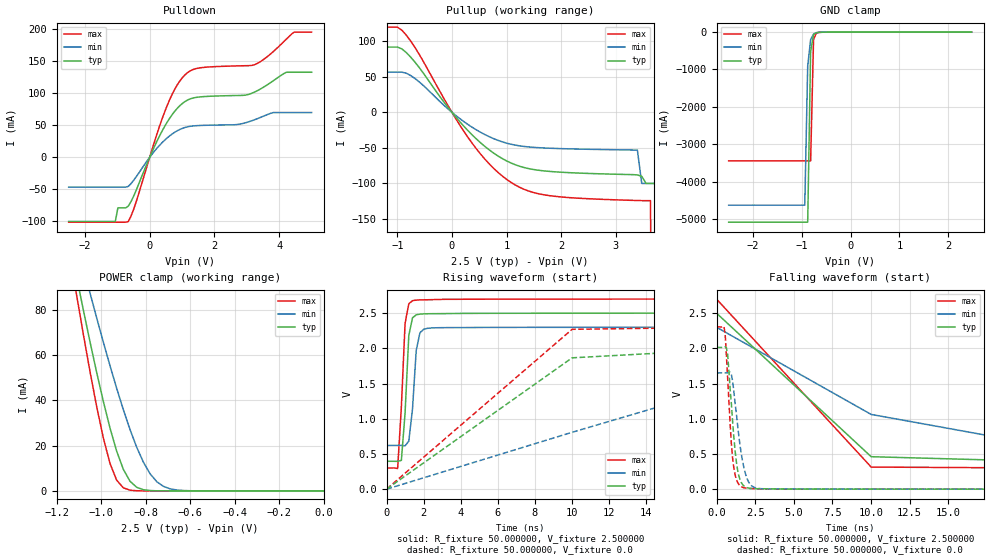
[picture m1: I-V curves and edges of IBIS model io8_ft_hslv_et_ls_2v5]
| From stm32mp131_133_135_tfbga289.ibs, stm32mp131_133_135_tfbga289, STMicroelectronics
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|   Model io8_ft_hslv_et_ls_2v5
[Model]  io8_ft_hslv_et_ls_2v5
Model_type I/O
Polarity   Non-Inverting
Enable   Active-Low
Vinl =   0.750000V
Vinh =   1.750000V
Vmeas =  1.250000V
Cref =   50.000000pF
Rref =   100.000000M
Vref =   0.0V
C_comp   3.268600pF   3.267200pF   3.310300pF
[Temperature Range]   25.000000   0.140000k   -40.000000
[Pullup Reference]   2.500000V   2.300000V   2.700000V
[Pulldown Reference]   0.0V   0.0V   0.0V
[POWER Clamp Reference]   2.500000V   2.300000V   2.700000V
[GND Clamp Reference]   0.0V   0.0V   0.0V
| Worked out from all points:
|   slope of the pulldown table from 0 to 0.375 V, typ, clamps not added: 9.35 ohm
|   slope of the pullup table from 0 to 0.375 V, typ, clamps not added: 11.7 ohm
|   GND clamp passes 1 mA (typ) near -0.47 V on its own axis
|   POWER clamp passes 1 mA (typ) near -0.82 V on its own axis
|   rising waveform, R_fixture 50.000000, V_fixture 2.500000: 20-80 % time 261ps typ, 279ps min, 266ps max; typ from 0.396 V to 2.5 V
|   rising waveform, R_fixture 50.000000, V_fixture 0.0: 20-80 % time 6.48ns typ, 12.5ns min, 6.1ns max; typ from 0 V to 2.01 V
|   falling waveform, R_fixture 50.000000, V_fixture 2.500000: 20-80 % time 6.2ns typ, 9.95ns min, 6.04ns max; typ from 2.5 V to 0.396 V
|   falling waveform, R_fixture 50.000000, V_fixture 0.0: 20-80 % time 452ps typ, 595ps min, 380ps max; typ from 2.01 V to 0 V
[Pulldown]
|Voltage   I(typ)   I(min)   I(max)
-2.5V     -100mA     -46.5mA    -101.2mA
-1.06V    -100mA     -46.5mA    -101.2mA
-980mV    -78.83mA   -46.5mA    -101.2mA
-660mV    -76.17mA   -45.35mA   -100.2mA
-420mV    -51.93mA   -30.73mA   -70.08mA
540mV     54.77mA    30.24mA    80.67mA
860mV     76.84mA    41.64mA    113.6mA
1.18V     89.58mA    47.73mA    132.5mA
3.26V     102.3mA    59.01mA    144.9mA
4.22V     132.7mA    69.88mA    184.3mA
4.46V     132.7mA    69.88mA    195.3mA
5V        132.7mA    69.88mA    195.3mA
[Pullup]
|Voltage   I(typ)   I(min)   I(max)
-2.5V     91.78mA    56.49mA    119.8mA
-920mV    89.28mA    56.49mA    115.6mA
-680mV    70.73mA    47.66mA    91.43mA
440mV     -36.9mA    -24.31mA   -50.57mA
840mV     -61.19mA   -39.29mA   -84.16mA
1.24V     -75.8mA    -47.13mA   -105.4mA
1.88V     -83.59mA   -50.71mA   -118mA
3.4V      -88mA      -53mA      -124mA
3.48V     -90mA      -100mA     -124.1mA
3.64V     -100mA     -100mA     -124.1mA
3.72V     -100mA     -100mA     -1A
4.92V     -100mA     -100mA     -1A
[GND_clamp]
|Voltage   I(typ)   I(min)   I(max)
-2.5V     -5.082A    -4.628A    -3.442A
-940mV    -5.082A    -4.628A    -3.442A
-880mV    -5.082A    -910.9mA   -3.442A
-820mV    -518.2mA   -200mA     -3.442A
-760mV    -65.41mA   -52.42mA   -196.1mA
-700mV    -14.98mA   -16.7mA    -21.53mA
-640mV    -6.913mA   -6.897mA   -7.503mA
2.48V     0A         42.99nA    0A
[POWER_clamp]
|Voltage   I(typ)   I(min)   I(max)
-2.49V    840.6mA    685.1mA    983.2mA
-1.11V    94.66mA    110.3mA    86.66mA
-1.08V    80.16mA    98.83mA    69.45mA
-1.05V    66.06mA    87.6mA     52.92mA
-990mV    39.64mA    65.82mA    23.5mA
-960mV    27.85mA    55.39mA    12.18mA
-930mV    17.59mA    45.37mA    4.744mA
-870mV    4.273mA    27.14mA    331.7uA
-810mV    535.4uA    12.72mA    17.14uA
-750mV    53.58uA    4.101mA    867.4nA
-630mV    505.3nA    181.4uA    0A
0V        0A         61.21nA    0A
[Ramp]
| variable   typ   min   max
dV/dt_r  1.20762/3.84208n   0.99054/6.91650n   1.38258/2.66491n
dV/dt_f  1.26240/2.45101n   1.00775/4.68867n   1.43924/1.72006n
R_load = 50.000000
[Rising Waveform]
R_fixture= 50.000000
V_fixture= 2.500000
V_fixture_min= 2.300000
V_fixture_max= 2.700000
|time   V(typ)   V(min)   V(max)
0s        396mV      620.4mV    301.3mV
600.6ps   394.8mV    620.4mV    293.7mV
800.8ps   409.1mV    621mV      1.169V
1.001ns   1.084V     616mV      2.355V
1.201ns   2.182V     681.5mV    2.633V
1.401ns   2.433V     1.14V      2.677V
1.602ns   2.476V     1.97V      2.685V
2.002ns   2.49V      2.27V      2.689V
3.003ns   2.493V     2.294V     2.696V
99.7ns    2.5V       2.3V       2.7V
[Rising Waveform]
R_fixture= 50.000000
V_fixture= 0.0
V_fixture_min= 0.0
V_fixture_max= 0.0
|time   V(typ)   V(min)   V(max)
0s        2.078nV    303.8nV    1.128nV
10.01ns   1.865V     807.7mV    2.271V
20.02ns   2.008V     1.584V     2.304V
30.03ns   2.013V     1.641V     2.304V
50.05ns   2.013V     1.651V     2.304V
991ns     2.013V     1.651V     2.304V
[Falling Waveform]
R_fixture= 50.000000
V_fixture= 2.500000
V_fixture_min= 2.300000
V_fixture_max= 2.700000
|time   V(typ)   V(min)   V(max)
0s        2.5V       2.3V       2.7V
10.01ns   461.1mV    1.062V     313.8mV
20.02ns   400.7mV    664.1mV    301.7mV
30.03ns   396.5mV    629.3mV    301.3mV
40.04ns   396.1mV    622.6mV    301.3mV
991ns     396mV      620.4mV    301.3mV
[Falling Waveform]
R_fixture= 50.000000
V_fixture= 0.0
V_fixture_min= 0.0
V_fixture_max= 0.0
|time   V(typ)   V(min)   V(max)
0s        2.013V     1.651V     2.304V
480.5ps   2.013V     1.651V     2.311V
640.6ps   2.009V     1.651V     1.895V
961ps     1.214V     1.626V     649.3mV
1.121ns   736.4mV    1.389V     301.1mV
1.361ns   275.3mV    916.4mV    98.01mV
1.762ns   47.88mV    316.4mV    20.93mV
2.242ns   9.89mV     53.26mV    9.068mV
3.043ns   5.98mV     5.006mV    3.057mV
39.88ns   2.078nV    303.8nV    1.128nV
